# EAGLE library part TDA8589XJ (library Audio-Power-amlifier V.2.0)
I2C-bus controlled 4 ´ 45 Watt power amplifier and multiple voltage regulator
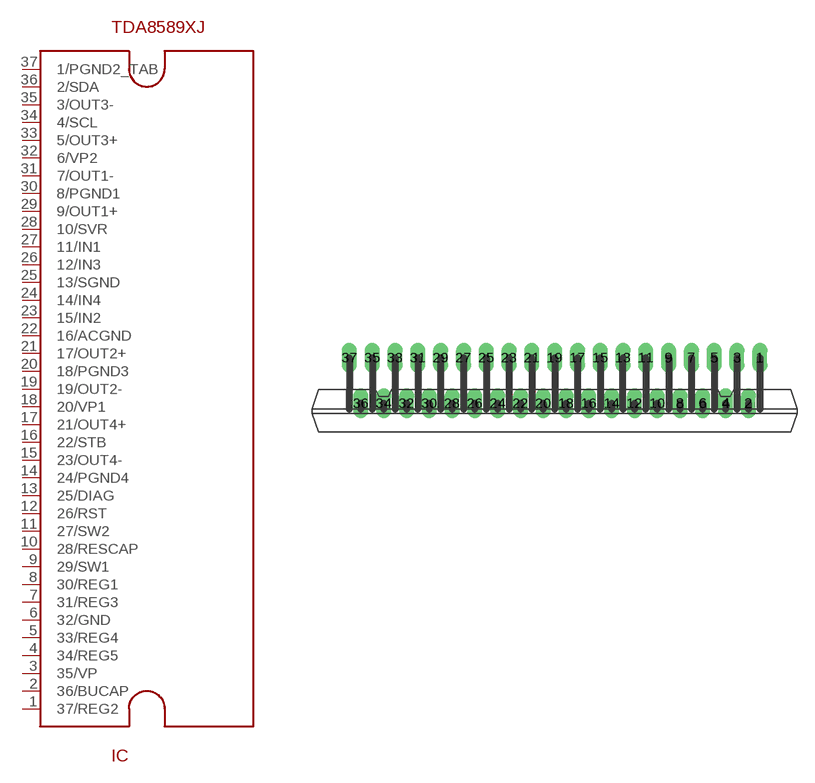
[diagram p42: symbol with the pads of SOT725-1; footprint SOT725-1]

Designator prefix IC

## TDA8589XJ  [SOT725-1]
1  37/REG2
2  36/BUCAP
3  35/VP  pwr
4  34/REG5
5  33/REG4
6  32/GND  pwr
7  31/REG3
8  30/REG1
9  29/SW1
10  28/RESCAP
11  27/SW2
12  26/RST
13  25/DIAG
14  24/PGND4  pwr
15  23/OUT4-  out
16  22/STB
17  21/OUT4+  out
18  20/VP1  pwr
19  19/OUT2-  out
20  18/PGND3  pwr
21  17/OUT2+  out
22  16/ACGND  pwr
23  15/IN2  in
24  14/IN4  in
25  13/SGND  pwr
26  12/IN3  in
27  11/IN1  in
28  10/SVR
29  9/OUT1+  out
30  8/PGND1  pwr
31  7/OUT1-  out
32  6/VP2  pwr
33  5/OUT3+  out
34  4/SCL
35  3/OUT3-  out
36  2/SDA
37  1/PGND2_TAB  pwr

## Footprint SOT725-1 (pad centres in mm)
drill 0.8 long: 1 18,4; 2 17,0; 3 16,4; 4 15,0; 5 14,4; 6 13,0; 7 12,4; 8 11,0; 9 10,4; 10 9,0; 11 8,4; 12 7,0; 13 6,4; 14 5,0; 15 4,4; 16 3,0; 17 2,4; 18 1,0; 19 0,4; 20 -1,0; 21 -2,4; 22 -3,0; 23 -4,4; 24 -5,0; 25 -6,4; 26 -7,0; 27 -8,4; 28 -9,0; 29 -10,4; 30 -11,0; 31 -12,4; 32 -13,0; 33 -14,4; 34 -15,0; 35 -16,4; 36 -17,0; 37 -18,4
